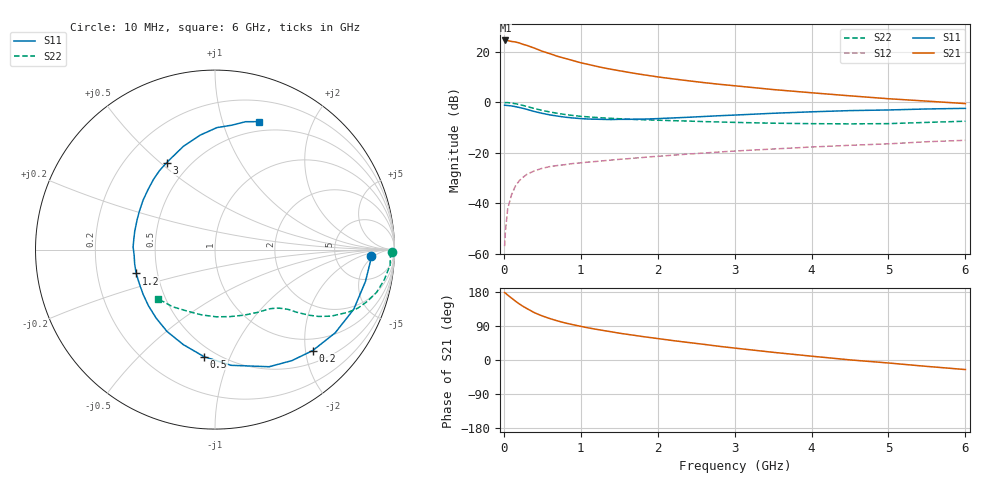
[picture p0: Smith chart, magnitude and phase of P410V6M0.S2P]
! SIEMENS Small Signal Semiconductors
! BFP182
! Si NPN RF Bipolar Junction Transistor in SOT143
! VCE = 10 V  IC = 6 mA
! Common Emitter S-Parameters:  March  1996
# GHz  S  MA  R  50
!  f  S11  S21  S12  S22
! GHz  MAG  ANG  MAG  ANG  MAG  ANG  MAG  ANG
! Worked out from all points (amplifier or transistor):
!   36 points, 10 MHz to 6 GHz, reference 50 ohm
!   highest |S21| = 24.4 dB at 20 MHz (marker M1)
!   |S21| within 3 dB of that: start of sweep to 393.5 MHz
!   unconditionally stable (mu >= 1): 1.593 GHz to 5.935 GHz
!   at 250 MHz: K = 0.22, MSG = 26.3 dB, |S12| = -29.8 dB
!   at 1.4 GHz: K = 0.94, MSG = 18.0 dB, |S12| = -22.9 dB
!   at 6 GHz: K = 0.99, MSG = 7.3 dB, |S12| = -15.1 dB
!   S11 on the Smith chart (normalised r, x): 10 MHz: 13, -4; 200 MHz: 0.74, -2.15; 500 MHz: 0.43, -0.81; 1.2 GHz: 0.38, -0.13; 3 GHz: 0.38, +0.52; 6 GHz: 0.40, +1.32
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0.01  0.8678 -2.2  16.52 177.9  0.0014 78.0  0.9854 -0.9
0.02  0.8673 -4.8  16.68 176.7  0.0027 88.0  0.9781 -2.0
0.05  0.8568 -12.0  16.59 171.3  0.0077 83.8  0.9792 -5.1
0.15  0.8145 -34.7  15.57 155.4  0.0217 70.6  0.9314 -14.8
0.2  0.783 -45.9  14.89 148.1  0.0276 65.8  0.8963 -18.8
0.25  0.7524 -55.3  13.96 141.5  0.0325 62.3  0.86 -22.3
0.3  0.7189 -65.2  13.3 135.7  0.0371 58.0  0.8199 -25.2
0.4  0.6509 -82.1  11.71 124.6  0.0437 51.8  0.7461 -29.8
0.5  0.5998 -95.8  10.19 116.2  0.0489 46.7  0.6857 -32.9
0.6  0.5579 -108.5  9.102 109.2  0.0529 43.9  0.6386 -34.9
0.7  0.5286 -120.4  8.079 103.0  0.0556 41.6  0.5993 -36.4
0.8  0.5031 -130.7  7.333 97.6  0.0578 39.7  0.5682 -37.7
1.1  0.4621 -156.0  5.581 84.7  0.065 37.3  0.5099 -40.4
1.2  0.4589 -163.2  5.145 81.1  0.0668 36.7  0.4973 -41.3
1.5  0.4566 178.1  4.196 70.8  0.0735 36.1  0.4689 -44.2
1.7  0.4587 167.1  3.717 65.0  0.0778 35.9  0.4531 -46.5
2.2  0.4863 145.5  2.888 51.2  0.0889 34.8  0.4293 -53.2
3  0.5543 119.1  2.111 31.5  0.1074 31.6  0.3971 -67.2
3.5  0.6015 107.1  1.777 20.3  0.1178 28.8  0.3825 -77.5
4.5  0.6797 89.1  1.333 0.3  0.1395 23.0  0.3712 -101.4
5.5  0.7324 76.6  1.047 -16.9  0.1643 17.5  0.3968 -126.7
6  0.7532 71.2  0.936 -25.2  0.1752 13.5  0.4185 -139.0
